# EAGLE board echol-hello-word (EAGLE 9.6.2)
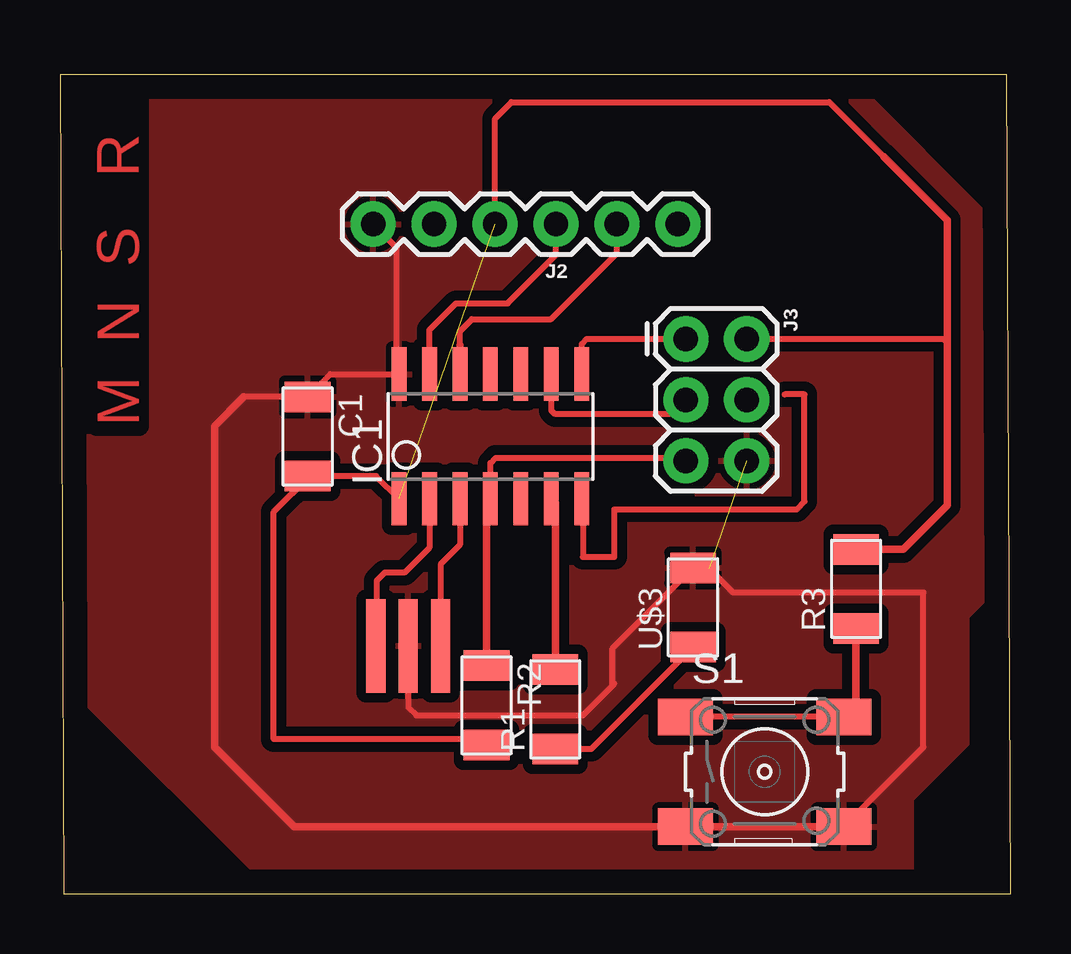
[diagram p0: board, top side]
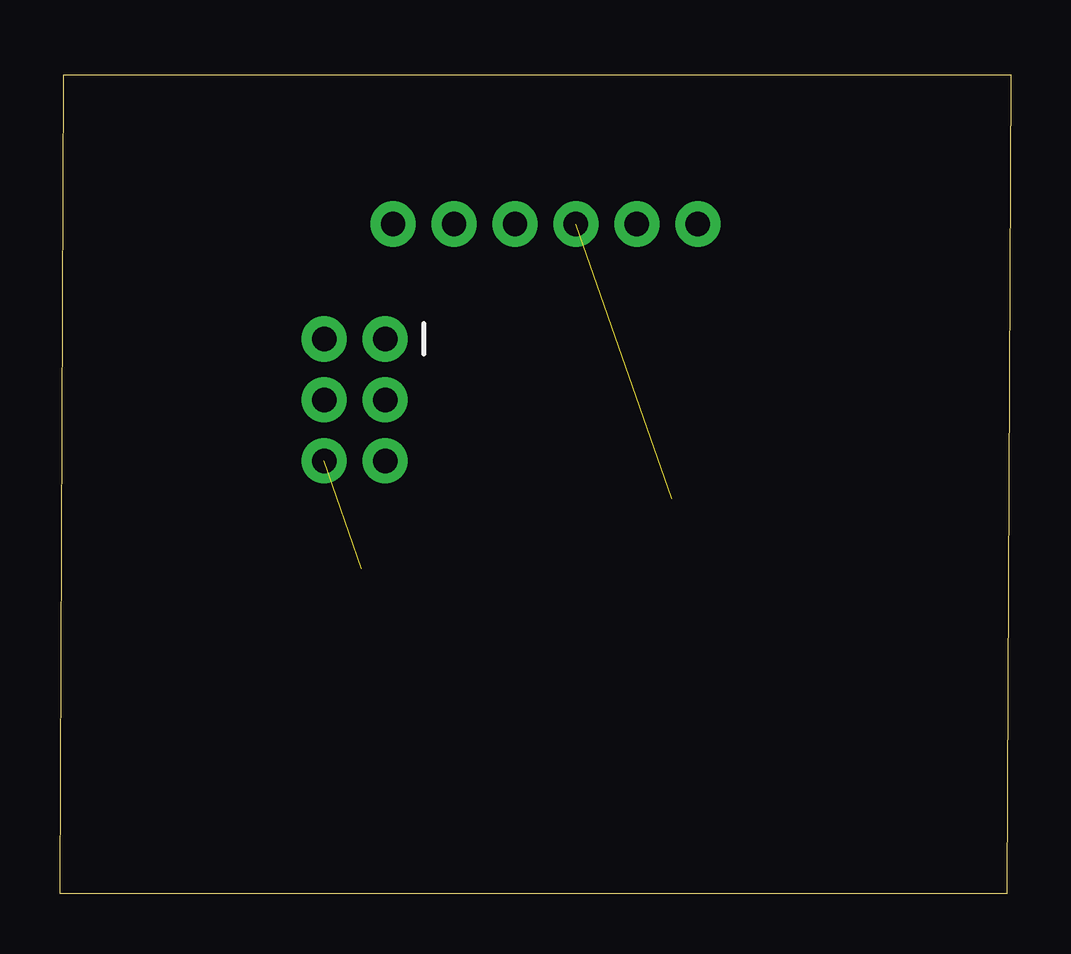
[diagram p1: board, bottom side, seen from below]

Size 39.64 x 34.13 mm. Coordinates in mm from the lower left corner, seen from the top.
Outline: 0.17,0 39.64,0 39.48,34.12 0,34.12 0.17,0
Copper layers (1*16): Top 0.035mm / dielectric 1.5mm / Bottom 0.035mm
Design rules "default": minimum track width 10mil, minimum drill 24mil, track to track 8mil, track to pad 8mil, pad to pad 8mil, via to via 8mil, smd to smd 8mil, copper to edge 40mil, drill to drill 8mil, minimum pad ring 10mil, minimum via ring 8mil, stop-mask expansion 4mil, vias tented up to drill 0mil, thermal gap 10mil

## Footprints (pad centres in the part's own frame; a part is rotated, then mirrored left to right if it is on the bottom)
C1206FAB = smd 1.27 x 1.905: 1 -1.651,0; 2 1.651,0
SOIC14 = smd 0.61 x 2.21: 1 -3.81,-2.603; 2 -2.54,-2.603; 3 -1.27,-2.603; 4 0,-2.603; 5 1.27,-2.603; 6 2.54,-2.603; 7 3.81,-2.603; 8 3.81,2.603; 9 2.54,2.603; 10 1.27,2.603; 11 0,2.603; 12 -1.27,2.603; 13 -2.54,2.603; 14 -3.81,2.603
FTDI_BASIC = drill 1.016 pad 1.88: CTS 10.16,0; DTR 0,0; GND 12.7,0; RXI 2.54,0; TXO 5.08,0; VCC 7.62,0
2X3 = drill 1.016 pad 1.88: 1 0,0; 2 0,2.54; 3 2.54,0; 4 2.54,2.54; 5 5.08,0; 6 5.08,2.54
R1206FAB = smd 1.27 x 1.905: 1 -1.651,0; 2 1.651,0
6MM_SWITCH = smd 2.286 x 1.524: 1 -3.302,2.286; 2 3.302,2.286; 3 -3.302,-2.286; 4 3.302,-2.286
EFOBM = smd 0.8 x 3.9: 1 -1.35,0; 2 0,0; 3 1.35,0
LED1206FAB = smd 1.27 x 1.905: 1 -1.651,0; 2 1.651,0

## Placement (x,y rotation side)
C1  1UF  [C1206FAB]  10.33,19.05 270 top
IC1  ATTINY44-SSU  [SOIC14]  17.95,19.05 0 top
J2  6_PIN_SERIAL_CABLEPTH  [FTDI_BASIC]  25.76,27.9 180 top
J3  [2X3]  26.09,23.11 270 top
R1  100  [R1206FAB]  20.65,7.68 90 top
R2  10k  [R1206FAB]  17.78,7.85 270 top
R3  10k  [R1206FAB]  33.19,12.7 90 top
S1  [6MM_SWITCH]  29.38,5.08 0 top
U$1  RESONATOR  [EFOBM]  14.52,10.33 0 top
U$3  LEDFAB1206  [LED1206FAB]  26.39,11.93 90 top

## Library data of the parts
C1 IC1 R1-R3 S1 U$1 U$3 = fab
J2 = SparkFun-Connectors
J3 = SparkFun-Connectors; PROD_ID: CONN-09701

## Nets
GND: C1.1 IC1.14 J2.GND J3.6 S1.3 S1.4 U$1.2 U$3.2
LED: IC1.6 R1.2
MISO: IC1.8 J3.1
MOSI: IC1.7
MOST: J3.4
N$1: R1.1 U$3.1
N$2: IC1.2 U$1.1
N$3: IC1.3 U$1.3
N$5: R3.1 S1.1 S1.2
RST: IC1.4 J3.5 R2.1
RXD: IC1.12 J2.RXI
SCK: IC1.9 J3.3
TXD: IC1.13 J2.TXO
VCC: C1.2 IC1.1 J2.VCC J3.2 R2.2 R3.2

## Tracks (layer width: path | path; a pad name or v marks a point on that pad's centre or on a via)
GND  (1 unrouted)
  Top 0.254: 7.66,20.7 C1.1 11.28,21.65 IC1.14 | 14.03,22.45 14.03,26.92 J2.GND | U$1.2 14.52,7.77 14.86,7.43 21.79,7.43 23.03,8.67 | 23.03,8.67 23.11,8.75 | S1.4 35.99,6.11 35.99,12.55 31.7,12.55 | 31.7,12.55 31.53,12.55 | 23.03,8.67 23.03,10.22 U$3.2 | 31.7,12.55 | 31.7,12.55 28.07,12.55 27.08,13.54
  Top 0.305: 7.66,20.7 6.44,19.48 6.44,6.11 9.75,2.79 S1.3 S1.4
  pour Top (isolate 0.406): 0.5,33.02 0.5,8.59 8.75,0.33 34.84,0.33 35.5,0.99 35.5,3.96 37.81,6.27 37.81,11.56 39.13,12.88 39.13,27.74 32.85,34.01 1.16,34.01 0.5,33.35
LED
  Top 0.305: IC1.6 20.65,16.28 R1.2
MISO
  Top 0.254: IC1.8 21.76,22.91 21.96,23.11 J3.1
MOSI
  Top 0.254: IC1.7 21.79,16.41 21.79,14.03 23.11,14.03 23.11,16.02 30.71,16.02 31.04,16.34 31.04,20.8 30.21,20.8
N$1
  Top 0.254: U$3.1 22.15,6.03 R1.1
N$2
  Top 0.254: IC1.2 15.41,14.41 14.36,13.37 13.54,13.37 13.21,13.04 13.21,10.37 U$1.1
N$3
  Top 0.254: IC1.3 16.68,14.53 15.87,13.72 15.87,11.56
  Top 0.305: U$1.3 15.87,11.56 15.87,11.68
N$5
  Top 0.254: S1.2 S1.1
  Top 0.305: S1.2 33.19,7.87 R3.1
RST
  Top 0.254: IC1.4 17.95,17.95 18.16,18.16 25.96,18.16 J3.5
  Top 0.305: R2.1 17.78,16.28 IC1.4
RXD
  Top 0.254: IC1.12 16.68,23.44 17.17,23.94 20.47,23.94 23.22,26.68 J2.RXI
  Top 0.305: IC1.12 16.68,22.86
SCK
  Top 0.254: J3.3 25.49,19.98 20.64,19.98 20.49,20.13 IC1.9
TXD
  Top 0.254: IC1.13 15.41,23.5 16.51,24.6 18.66,24.6 20.68,26.62 J2.TXO
VCC  (1 unrouted)
  Top 0.254: 34.34,30.71 32.07,32.98 18.82,32.98 18.14,32.3 J2.VCC | J3.2 36.82,23.11 36.98,22.95 | C1.2 10.4,17.4 | 10.4,17.4 13.18,17.4 IC1.1 | R2.2 17.54,6.44 8.92,6.44 8.92,15.91 10.4,17.4
  Top 0.305: 33.19,14.2 R3.2 35.15,14.35 36.98,16.18 36.98,22.95 36.98,28.07 34.34,30.71 | 17.83,6.15 R2.2

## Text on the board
Top: M N S R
